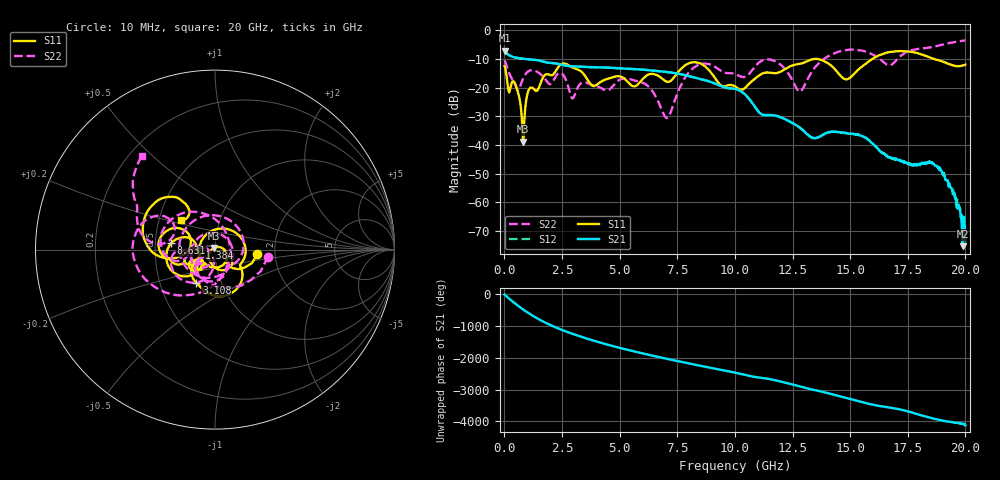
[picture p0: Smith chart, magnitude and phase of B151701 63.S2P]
!  2-Port S-parameters saved by WinCal
! VAR MeasName=S-Parameters (CALIBRATED_DATA) read from VNA (N5244A)
! VAR MeasDate=2015-12-24 19:17:25
! VAR NAME=B151701 63
! VAR FILENAME=B151701 63.S2P
! VAR DATE=2015-12-24 19:17:25
! VAR PHYS_PORTS=1,3
# Hz S DB R 50
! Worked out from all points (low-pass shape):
!   801 points, 10 MHz to 20 GHz, reference 50 ohm
!   highest |S21| = -7.13 dB at 10 MHz (marker M1); lowest = -75.3 dB at 19.88 GHz (marker M2)
!   |S21| within 3 dB of the highest: start of sweep to 987 MHz
!   lowest |S11| = -38.8 dB at 809.6 MHz (marker M3), VSWR 1.02, Z = 49.3 + j0.86 ohm
!   |S11| at or under -10 dB: start of sweep to 15.97 GHz; 18.63 GHz to end of sweep
!   |S22| runs from -30.6 to -3.6 dB; largest |S21 - S12| = 0.0023
!   S11 on the Smith chart (normalised r, x): 10 MHz: 1.61, -0.09; 1.384 GHz: 0.84, +0.01; 3.108 GHz: 0.76, -0.30; 8.631 GHz: 0.61, +0.05; 20 GHz: 0.65, +0.22
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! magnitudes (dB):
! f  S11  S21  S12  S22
! 10 MHz  -12.5  -7.1  -7.1  -10.5
! 509.8 MHz  -19.6  -9.6  -9.6  -19.9
! 809.6 MHz  -38.8  -9.9  -9.9  -16.9
! 1.059 GHz  -20.8  -10.2  -10.2  -14.2
! 1.384 GHz  -21.2  -10.4  -10.4  -14.3
! 2.484 GHz  -11.8  -12.1  -12.1  -15.1
! 3.108 GHz  -13.5  -12.6  -12.6  -21.3
! 3.358 GHz  -14.6  -12.8  -12.8  -18.3
! 5.432 GHz  -18.7  -13.5  -13.5  -17.0
! 6.682 GHz  -16.0  -14.3  -14.3  -25.0
! 7.106 GHz  -18.0  -14.6  -14.6  -30.4
! 7.881 GHz  -12.0  -15.8  -15.8  -16.0
! 8.631 GHz  -12.2  -17.3  -17.3  -11.7
! 10.01 GHz  -19.6  -20.5  -20.4  -15.3
! 11.58 GHz  -14.9  -29.6  -29.6  -10.4
! 12.8 GHz  -11.7  -33.9  -33.9  -21.4
! 13.35 GHz  -10.2  -37.4  -37.5  -14.3
! 14.85 GHz  -17.2  -35.8  -35.9  -6.9
! 16.68 GHz  -7.7  -44.4  -44.3  -12.3
! 18.8 GHz  -10.4  -47.6  -47.5  -5.5
! 19.88 GHz  -12.3  -75.3  -64.4  -3.7
! 20 GHz  -12.0  -73.1  -70.7  -3.6
